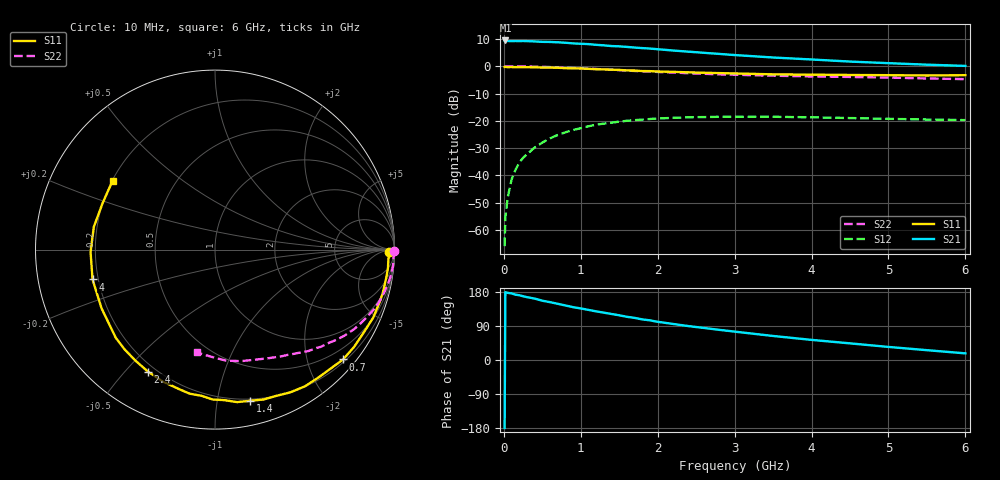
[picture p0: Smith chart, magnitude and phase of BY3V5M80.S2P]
! SIEMENS Small Signal Semiconductors
! BFY420
! Si NPN RF SIEGET Grounded Emitter Transistor in MICRO-X
! VCE = 3.5 V  IC = 0.8 mA
! Common Emitter S-Parameters:  October  1996
# GHz  S  MA  R  50
!  f  S11  S21  S12  S22
! GHz  MAG  ANG  MAG  ANG  MAG  ANG  MAG  ANG
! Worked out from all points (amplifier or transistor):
!   36 points, 10 MHz to 6 GHz, reference 50 ohm
!   highest |S21| = 9.5 dB at 20 MHz (marker M1)
!   |S21| within 3 dB of that: start of sweep to 1.913 GHz
!   unconditionally stable (mu >= 1): 4.623 GHz to end of sweep
!   at 250 MHz: K = 0.05, MSG = 21.4 dB, |S12| = -33.6 dB
!   at 1.4 GHz: K = 0.17, MSG = 14.1 dB, |S12| = -20.7 dB
!   at 6 GHz: K = 1.37, MAG = 6.3 dB, |S12| = -19.7 dB
!   S11 on the Smith chart (normalised r, x): 10 MHz: 59, -25; 700 MHz: 0.25, -2.68; 1.4 GHz: 0.19, -1.24; 2.4 GHz: 0.17, -0.58; 4 GHz: 0.18, -0.12; 6 GHz: 0.20, +0.29
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0.01  0.9716 -0.7  2.959 -179.4  0.0005 86.4  0.9983 -0.3
0.02  0.9751 -1.3  2.981 178.8  0.0017 89.5  0.9977 -0.5
0.05  0.9675 -3.0  2.911 177.2  0.0039 89.4  0.9982 -1.3
0.1  0.969 -5.9  2.904 175.8  0.0083 84.9  0.9958 -2.7
0.15  0.9673 -8.8  2.91 172.4  0.0125 82.9  0.9963 -4.0
0.2  0.9655 -11.8  2.9 171.0  0.0169 82.3  0.9957 -5.3
0.3  0.9631 -17.5  2.901 165.9  0.0243 79.7  0.9915 -8.0
0.4  0.9594 -23.3  2.862 162.1  0.0323 76.0  0.9843 -10.6
0.5  0.9486 -29.2  2.812 156.5  0.0398 72.7  0.9761 -13.2
0.7  0.9402 -40.6  2.759 148.3  0.0549 65.6  0.9567 -18.3
0.9  0.9161 -51.4  2.633 139.5  0.0677 58.7  0.9313 -23.0
1.1  0.8992 -62.2  2.554 132.2  0.0793 52.9  0.9056 -27.6
1.4  0.865 -76.8  2.353 121.4  0.0923 44.3  0.8655 -33.7
1.8  0.8179 -95.3  2.158 107.2  0.1052 34.4  0.8115 -40.7
2.2  0.7903 -111.7  1.948 95.1  0.1134 25.9  0.7686 -47.3
2.4  0.7755 -118.8  1.857 89.5  0.116 22.5  0.7458 -50.2
2.8  0.7503 -132.1  1.689 79.6  0.1184 16.2  0.7117 -55.6
3.5  0.7117 -152.7  1.451 63.4  0.1185 7.8  0.6728 -64.2
4  0.7023 -166.3  1.334 53.1  0.1159 3.7  0.6513 -70.5
4.5  0.6934 -178.8  1.221 43.9  0.1123 0.5  0.638 -77.0
5.5  0.6777 157.3  1.071 25.9  0.1055 -1.5  0.598 -91.8
6  0.6874 146.0  1.017 17.5  0.1031 -0.4  0.5817 -100.2
